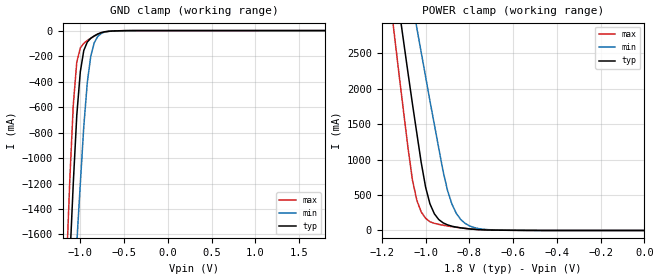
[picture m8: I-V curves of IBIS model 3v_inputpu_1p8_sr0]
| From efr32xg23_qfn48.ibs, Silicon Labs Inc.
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|   Model 3v_inputpu_1p8_sr0
[Model]  3v_inputpu_1p8_sr0
Model_type Input
C_comp   1.6300pF   1.4000pF   2.7000pF
[Temperature Range]   25.0000   0.1250k   -40.0000
[Pullup Reference]   1.8000V   1.6200V   1.9800V
[Pulldown Reference]   0.0V   0.0V   0.0V
[POWER Clamp Reference]   1.8000V   1.6200V   1.9800V
[GND Clamp Reference]   0.0V   0.0V   0.0V
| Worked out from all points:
|   GND clamp passes 1 mA (typ) near -0.52 V on its own axis
|   POWER clamp passes 1 mA (typ) near -0.53 V on its own axis
[GND_clamp]
|Voltage   I(typ)   I(min)   I(max)
-1.8V     -14.24A    -14.11A    -14.46A
-1.16V    -2.476A    -3.328A    -1.893A
-1.12V    -1.809A    -2.723A    -1.176A
-1.08V    -1.199A    -2.174A    -584.6mA
-1.04V    -665.4mA   -1.671A    -246.3mA
-1V       -325.1mA   -1.206A    -136.5mA
-960mV    -156.4mA   -753.1mA   -99.71mA
-920mV    -90.26mA   -408.8mA   -78.11mA
-880mV    -60.46mA   -200mA     -59.79mA
-840mV    -41.42mA   -94.71mA   -43.18mA
-640mV    -3.854mA   -4.307mA   -4.163mA
1.8V      619.3pA    4.343uA    -4.631uA
[POWER_clamp]
|Voltage   I(typ)   I(min)   I(max)
-1.8V     20.85A     19.71A     22.07A
-1.16V    4.023A     5.096A     3.217A
-1.14V    3.56A      4.702A     2.691A
-1.1V     2.657A     3.938A     1.662A
-1.06V    1.784A     3.203A     710.9mA
-1.04V    1.371A     2.858A     425mA
-1V       612.4mA    2.171A     172.4mA
-980mV    375.2mA    1.828A     122.5mA
-900mV    79.37mA    567.6mA    63.71mA
-860mV    47.62mA    243.7mA    45.05mA
-820mV    29.32mA    101.5mA    29.66mA
0V        619.3pA    9.371nA    573.9pA
